
FUNCTION_BLOCK FB103

TITLE =   <Salida Analogica >
//
//   <Baustein-Kommentar/ Block comment>
//   Hier können Sie Informationen zu Ihrem Baustein hinterlegen
//   You can store information about your block here
//
//   statt FB<Baustein-Nr> kann auch <Name aus Symboltabelle> angegeben werden;
//   In place of FB<block no.>, <symbolic name> can also be entered;

AUTHOR:   Andy     //  max. 8 Zeichen / max. 8 characters
FAMILY:   plant1   //  max. 8 Zeichen / max. 8 characters
NAME:     fb_mot21 //  max. 8 Zeichen / max. 8 characters
VERSION:  01.01    //  max. 15.15
// KNOW_HOW_PROTECT
//   (falls angegeben, kann im generierten Baustein keine Änderungen mehr vorgenommen werden)
//   (If specified, no more changes can be made once the block is generated)
//
//   Die Vorbelegung von Variablen ist nur für INPUT-, OUTPUT-, IN_OUT-
//   und VAR- Variable möglich; nicht für VAR_TEMP.
//   Assigning variables is only possible for INPUT, OUTPUT, IN_OUT,
//   and VAR variables; not for VAR_TEMP

VAR_INPUT
  IN1: INT:=123;
END_VAR

VAR_OUTPUT
  OUT1: INT:=123;
END_VAR

VAR_IN_OUT
  IN_OUT1: INT:=123;
END_VAR

VAR
  VAR1: INT:=123;
END_VAR

VAR_TEMP
  TEMP1: INT;
END_VAR

BEGIN
NETWORK
TITLE =   <Überschrift von 1. Netzwerk/ Title of first network>
//
//  <Netzwerk-Kommentar/ Network comment>
//  Hier können Sie Informationen zu Ihrem Netzwerk hinterlegen
//  You can store information about your network here

//  Anweisungen des Netzwerks
//  z.B. FB-Aufruf:
//  CALL FB1, DB1
//    ( <Parameter-Name>:=<Aktualparameter>   ; weitere Parameter
//     );
//   Parameterübergaben sind beim FB optional, sie können einzeln oder gesamt
//   (incl. () ) weggelassen werden. Auch beim Aufruf kann statt FB bzw.
//   DB<Baustein-Nr> ein Name aus der Symboltabelle angegeben werden.

//  Instructions in the network
//  for example, FB call:
//  CALL FB1, DB1
//    ( <parameter name>:=<actual parameter>   ; additional parameters
//     );
//   Parameter passing is optional in the FB, individual parameters or the whole
//   parameter (including () ) can be left out. For the block call, you can also specify
//   a symbolic name from the symbol table instead of the FB or DB<block no.>.

//   Folge-Netzwerke/ Other networks


END_FUNCTION_BLOCK

